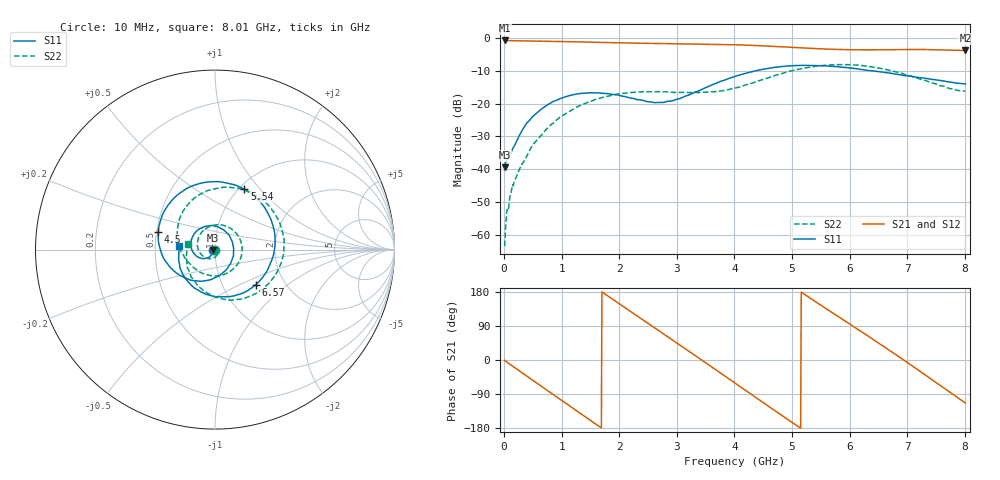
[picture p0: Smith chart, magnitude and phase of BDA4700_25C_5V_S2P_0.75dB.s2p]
!Agilent Technologies,E5071B,MY42404982,A.09.10
!Date: Mon Oct 20 13:26:19 2025
!Data & Calibration Information:
!Freq	S11:SOLT2(ON)	S21:SOLT2(ON)	S12:SOLT2(ON)	S22:SOLT2(ON)
# Hz S RI R 50
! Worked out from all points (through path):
!   801 points, 10 MHz to 8.01 GHz, reference 50 ohm
!   highest |S21| = -0.87 dB at 10 MHz (marker M1); lowest = -3.9 dB at 8.01 GHz (marker M2)
!   group delay of S21, straight-line fit = 288 ps
!   lowest |S11| = -39.3 dB at 10 MHz (marker M3), VSWR 1.02, Z = 49 - j0.227 ohm
!   |S11| at or under -10 dB: start of sweep to 4.383 GHz; 6.335 GHz to end of sweep
!   |S22| runs from -63.3 to -8.2 dB; largest |S21 - S12| = 0.0071
!   S11 on the Smith chart (normalised r, x): 10 MHz: 0.98, -0.00; 4.5 GHz: 0.51, +0.12; 5.54 GHz: 1.06, +0.83; 6.57 GHz: 1.43, -0.62; 8.01 GHz: 0.67, +0.03
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1e7  -0.0106 -0.00232  0.9046 -0.0195  0.9044 -0.0203  -0.000276 -0.000627
1.5e8  -0.0138 -0.0153  0.8603 -0.2526  0.8601 -0.2526  0.00319 0.00489
4.8e8  -0.0407 -0.0451  0.5517 -0.6942  0.5511 -0.6946  0.0169 -0.0142
9e8  -0.1062 -0.0334  -0.0921 -0.8691  -0.0918 -0.8691  -0.0225 -0.0503
1.35e9  -0.1317 0.054  -0.69 -0.5106  -0.6908 -0.5108  -0.0954 0.00705
1.92e9  -0.0281 0.1335  -0.7687 0.3298  -0.769 0.3302  -0.00787 0.136
2.32e9  0.0643 0.0944  -0.351 0.7436  -0.3512 0.7441  0.1182 0.0913
2.68e9  0.1034 0.0112  0.1686 0.7959  0.1688 0.7957  0.1478 -0.0321
3.06e9  0.0777 -0.091  0.6298 0.5007  0.6275 0.5032  0.068 -0.1307
3.36e9  0.00902 -0.1523  0.7913 0.1026  0.7925 0.1019  -0.0224 -0.1449
3.67e9  -0.0986 -0.1747  0.7151 -0.3342  0.7152 -0.336  -0.1009 -0.1128
4.01e9  -0.2272 -0.1208  0.3789 -0.6799  0.3794 -0.6794  -0.1625 -0.0534
4.5e9  -0.3159 0.1002  -0.2881 -0.6921  -0.2872 -0.6941  -0.2104 0.0981
4.92e9  -0.2031 0.3092  -0.658 -0.2877  -0.6579 -0.29  -0.1317 0.2729
5.35e9  0.0486 0.3745  -0.6434 0.2375  -0.6443 0.236  0.1026 0.3445
5.54e9  0.1632 0.3363  -0.5209 0.4263  -0.5213 0.4261  0.2183 0.3079
6.05e9  0.3341 0.0781  0.000293 0.6522  -0.000309 0.6548  0.3846 0.0334
6.57e9  0.2259 -0.1966  0.5173 0.4024  0.5181 0.4009  0.2369 -0.2395
6.68e9  0.1751 -0.2327  0.5854 0.2931  0.5872 0.2925  0.1803 -0.2649
7.23e9  -0.0891 -0.2291  0.5669 -0.3376  0.5671 -0.3385  -0.0698 -0.2225
7.62e9  -0.1915 -0.1103  0.1983 -0.62  0.1978 -0.6209  -0.154 -0.0999
8.01e9  -0.1981 0.0195  -0.2565 -0.5836  -0.2556 -0.5848  -0.1507 0.0318
